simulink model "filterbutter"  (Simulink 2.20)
settings: Solver=VariableStepDiscrete  StartTime=0.0  StopTime=23  RelTol=1e-3  AbsTol=1e-6
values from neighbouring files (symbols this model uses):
  a = input('Inserisci il dato da graficare [1=PIDNL 2=PD 3=PID]: ')    [grp.m]    (also in grp1.m = input('Inserisci il dato da graficare [1..3]'))
undefined symbols (not defined in the file or in its folder): b

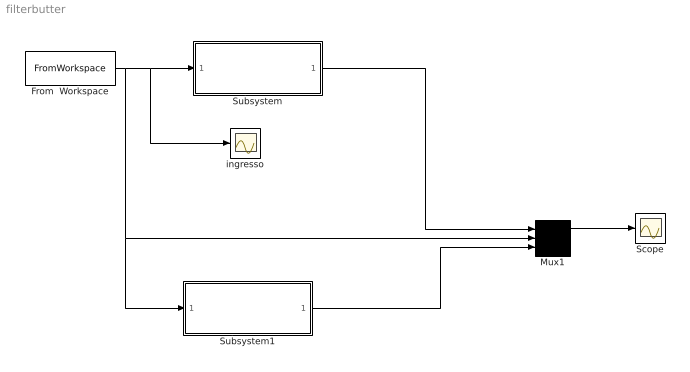
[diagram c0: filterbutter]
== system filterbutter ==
  From  Workspace : FromWorkspace  VariableName=[out(:,1),out(:,10)]
  Mux1 : Mux  Inputs=3
  Scope : Scope
  Subsystem : Subsystem  mask(Filtro di Butterworth){ordine=3, freq=0.2/16}
      mask prompts: ordine "Ordine del filtro"; freq "Parametro K per ricavare la Freq. di taglio Ft"
      mask help: Attenzione! Considerare il parametro Fc come la frequanza di campionamento del segnale di ingresso, per cui la frequanza di taglio diviene Ft=K*Fc;
      mask init:
      | [b,a]=butter(ordine,freq);
  Subsystem1 : Subsystem  mask(Filtro di Butterworth){ordine=5, freq=0.5/16}
      mask prompts: ordine "Ordine del filtro"; freq "Parametro K per ricavare la Freq. di taglio Ft"
      mask help: Attenzione! Considerare il parametro Fc come la frequanza di campionamento del segnale di ingresso, per cui la frequanza di taglio diviene Ft=K*Fc;
      mask init:
      | [b,a]=butter(ordine,freq);
  ingresso : Scope
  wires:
  From  Workspace/1 -> Mux1/2, Subsystem1/1(In1), Subsystem/1(In1), ingresso/1
  Mux1/1 -> Scope/1
  Subsystem/1(Out1) -> Mux1/1
  Subsystem1/1(Out1) -> Mux1/3

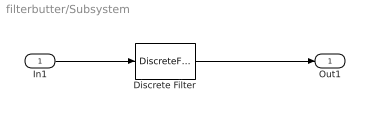
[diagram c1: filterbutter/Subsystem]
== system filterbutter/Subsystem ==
  In1 : Inport  Port=1  PortWidth=-1  SampleTime=-1
  Discrete Filter : DiscreteFilter  Numerator=b  Denominator=a  SampleTime=.032
  Out1 : Outport  Port=1
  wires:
  In1/1 -> Discrete Filter/1
  Discrete Filter/1 -> Out1/1

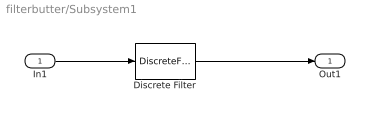
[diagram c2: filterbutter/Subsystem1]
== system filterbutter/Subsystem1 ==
  In1 : Inport  Port=1  PortWidth=-1  SampleTime=-1
  Discrete Filter : DiscreteFilter  Numerator=b  Denominator=a  SampleTime=.032
  Out1 : Outport  Port=1
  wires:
  In1/1 -> Discrete Filter/1
  Discrete Filter/1 -> Out1/1
